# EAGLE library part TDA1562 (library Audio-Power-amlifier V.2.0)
70 W High Efficiency Power Amplifier with diagnostic facility
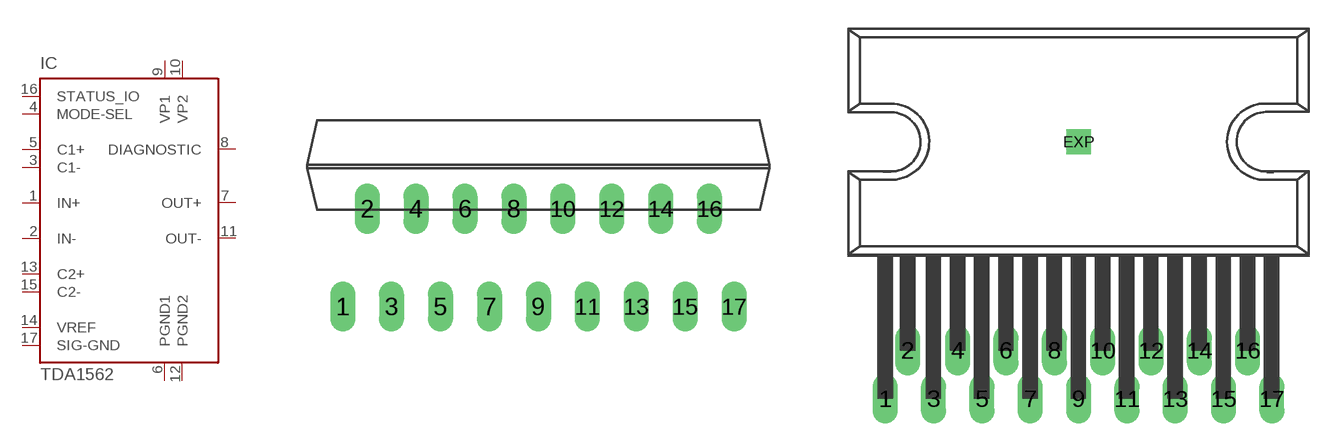
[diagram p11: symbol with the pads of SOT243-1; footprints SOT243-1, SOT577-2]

Designator prefix IC

## TDA1562TDA1562Q  [SOT243-1]
1  IN+  in
2  IN-  in
3  C1-  pas
4  MODE-SEL  in
5  C1+  pas
6  PGND1  pwr
7  OUT+  out
8  DIAGNOSTIC  out
9  VP1  pwr
10  VP2  pwr
11  OUT-  out
12  PGND2  pwr
13  C2+  pas
14  VREF  in
15  C2-  pas
16  STATUS_IO  in
17  SIG-GND  in

## TDA1562TDA1562ST  [SOT577-2]
Pads as for SOT243-1

## TDA1562TDA1562SD  [SOT668-2]
Pads as for SOT243-1

## Footprint SOT243-1 (pad centres in mm)
DBS17P: plastic DIL-bent-SIL power package; 17 leads (lead length 7.7 mm)
drill 0.8 long: 1 -10.16,-5.08; 2 -8.89,0; 3 -7.62,-5.08; 4 -6.35,0; 5 -5.08,-5.08; 6 -3.81,0; 7 -2.54,-5.08; 8 -1.27,0; 9 0,-5.08; 10 1.27,0; 11 2.54,-5.08; 12 3.81,0; 13 5.08,-5.08; 14 6.35,0; 15 7.62,-5.08; 16 8.89,0; 17 10.17,-5.08

## Footprint SOT577-2 (pad centres in mm)
drill 0.8 long: 1 -10.16,-13.5; 2 -8.98,-10.96; 3 -7.62,-13.5; 4 -6.35,-10.96; 5 -5.08,-13.5; 6 -3.81,-10.96; 7 -2.54,-13.5; 8 -1.27,-10.96; 9 0,-13.5; 10 1.27,-10.96; 11 2.54,-13.5; 12 3.81,-10.96; 13 5.08,-13.5; 14 6.35,-10.96; 15 7.62,-13.5; 16 8.89,-10.96; 17 10.16,-13.5
drill 0.8 square: EXP 0,0

## Footprint SOT668-2 (pad centres in mm)
RDBS17P: plastic rectangular-DIL-bent-SIL (reverse bent) power package; 17 leads (row spacing 2.54 mm)
drill 0.7 long: 1 -10.16,-5.08; 2 -8.89,-2.54; 3 -7.62,-5.08; 4 -6.35,-2.54; 5 -5.08,-5.08; 6 -3.81,-2.54; 7 -2.54,-5.08; 8 -1.27,-2.54; 9 0,-5.08; 10 1.27,-2.54; 11 2.54,-5.08; 12 3.81,-2.54; 13 5.08,-5.08; 14 6.35,-2.54; 15 7.62,-5.08; 16 8.89,-2.54; 17 10.16,-5.08
smd 10 x 6: EXP 0,8.42
hole 3.2 at -10,8.42
hole 3.2 at 10,8.42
